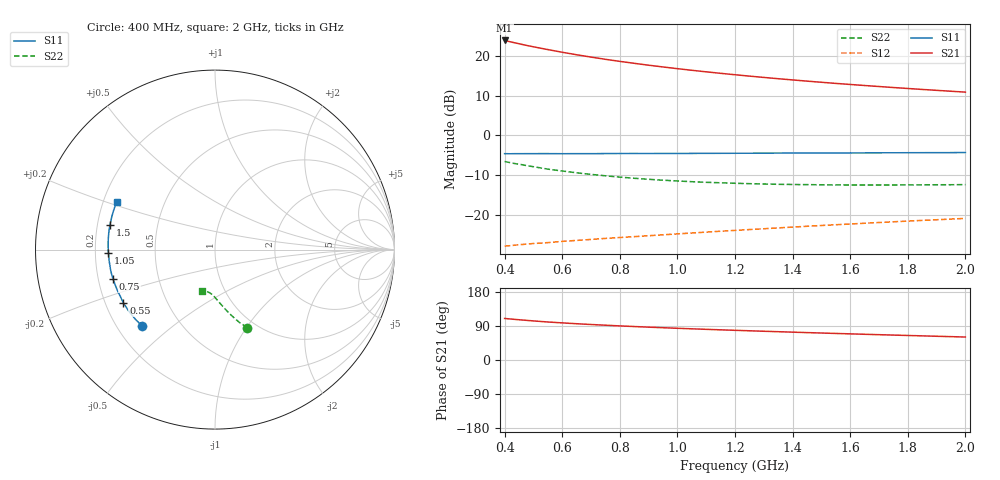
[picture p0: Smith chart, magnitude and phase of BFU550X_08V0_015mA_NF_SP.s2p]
! Filename:  P:\Prog\Test\Noise\ATS_data\Testdata_Net\BFU550X attenuator noise\BFU550X_APG2013_44_C05_08p0V_015mA_NF_CM01_D.sf
! Date/Time: Fri 26/Jul/2013 14:34:23
! BFU550X_APG2013_44_C05_08p0V_1to35mA_NF_CM01_Bias6_R.sf
! Noise Parameter Data File
! BFU550X_APG2013_44_C05_08p0V_1to35mA_NF_CM01
! Date/time: Mon Jul 22 10:19:05 2013
! VAR V_out= 8.001000
! VAR I_out= 14.995000
! VAR V_in= 0.808100
! VAR I_in= 0.159400
! Device data file deembeded for feedlines and parallel
! Original file: \BFU550X attenuator noise\BFU550X_APG2013_44_C05_08p0V_015mA_NF_CM01_R.sf
! Feed-files: PR005V01_100713_Feed1.s2p, PR005V01_100713_Feed2.s2p
! Parallel-file: PR005V01_100713_Par.s2p
# MHz S MA R 50
!  Freq-MHz  S11-mag  S11-arg  S21-mag  S21-arg  S12-mag  S12-arg  S22-mag  S22-arg
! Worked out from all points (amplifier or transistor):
!   37 points, 400 MHz to 2 GHz, reference 50 ohm
!   highest |S21| = 23.9 dB at 400 MHz (marker M1)
!   |S21| within 3 dB of that: start of sweep to 602.9 MHz
!   unconditionally stable (mu >= 1): 1.724 GHz to end of sweep
!   at 500 MHz: K = 0.53, MSG = 24.7 dB, |S12| = -27.2 dB
!   at 1.1 GHz: K = 0.86, MSG = 20.1 dB, |S12| = -24.3 dB
!   at 2 GHz: K = 1.03, MAG = 14.8 dB, |S12| = -20.9 dB
!   lowest NFmin = 0.92 dB at 420 MHz
!   S11 on the Smith chart (normalised r, x): 400 MHz: 0.30, -0.40; 550 MHz: 0.27, -0.25; 750 MHz: 0.26, -0.13; 1.05 GHz: 0.25, -0.02; 1.5 GHz: 0.25, +0.11; 2 GHz: 0.26, +0.22
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400  0.5893 -133.4  15.61 109.7  0.04052 44.7  0.4705 -67.6
420  0.5876 -135.8  15 108.2  0.04115 44.5  0.4541 -69.0
440  0.5892 -138.3  14.46 106.9  0.04188 44.2  0.4397 -70.1
460  0.5891 -140.6  13.93 105.6  0.04252 44.0  0.4287 -71.4
500  0.5902 -144.9  12.99 103.2  0.04375 43.7  0.4042 -73.5
550  0.5904 -149.8  11.99 100.3  0.04491 43.6  0.3769 -76.0
600  0.5886 -153.7  11.1 97.9  0.04651 43.9  0.3569 -78.1
650  0.5896 -157.5  10.32 95.7  0.04788 44.0  0.3388 -80.0
700  0.5897 -160.7  9.644 93.7  0.04924 44.3  0.3236 -81.7
750  0.5909 -163.7  9.047 91.8  0.05074 44.7  0.3105 -83.3
800  0.5922 -166.6  8.525 90.0  0.05205 45.0  0.2991 -84.9
850  0.5926 -169.2  8.054 88.3  0.05339 45.5  0.2891 -86.2
900  0.5921 -171.6  7.627 86.7  0.05482 46.0  0.2807 -87.5
950  0.5931 -173.9  7.248 85.2  0.05632 46.5  0.2735 -88.7
1050  0.5938 -178.0  6.583 82.3  0.05933 47.4  0.2618 -91.0
1100  0.5949 -180.0  6.294 80.9  0.06087 47.8  0.2573 -92.0
1200  0.5963 176.4  5.787 78.3  0.06397 48.5  0.2501 -94.0
1350  0.5989 171.4  5.159 74.7  0.06878 49.5  0.2428 -96.8
1500  0.601 166.9  4.654 71.2  0.07369 50.2  0.2394 -99.3
1600  0.6024 164.1  4.367 69.0  0.07695 50.5  0.238 -100.9
1750  0.6047 160.1  3.997 65.8  0.08207 51.0  0.2382 -103.3
2000  0.6091 154.0  3.5 60.6  0.0905 51.4  0.2407 -106.9
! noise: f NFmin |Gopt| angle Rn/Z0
400  1.005  0.1461  -178.7  0.0901
460  0.931  0.2236  -177.6  0.0677
600  0.9512  0.1997  -176.6  0.0789
800  0.9348  0.2347  -173.6  0.0744
1000  0.9968  0.2728  -176.7  0.0624
1200  1.026  0.2772  -175.9  0.0654
1400  1.043  0.3075  -171.9  0.0639
1600  1.094  0.3049  -163.1  0.0742
1800  1.108  0.3363  -169.6  0.0602
2000  1.144  0.3586  -166.1  0.067
